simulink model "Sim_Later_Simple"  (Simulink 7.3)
settings: Solver=ode45  StartTime=0.0  StopTime=20  RelTol=1e-3
InitFcn:
  | init
StartFcn:
  | init
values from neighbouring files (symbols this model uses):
  d2r = pi/180    (= 0.0174532925199)    [init.m]    (also in robust.m)
  r2d = 180/pi    (= 57.2957795131)    [init.m]    (also in robust.m)
undefined symbols (not defined in the file or in its folder): Als, Bls, Cls, Dls, Kmix, Kpr

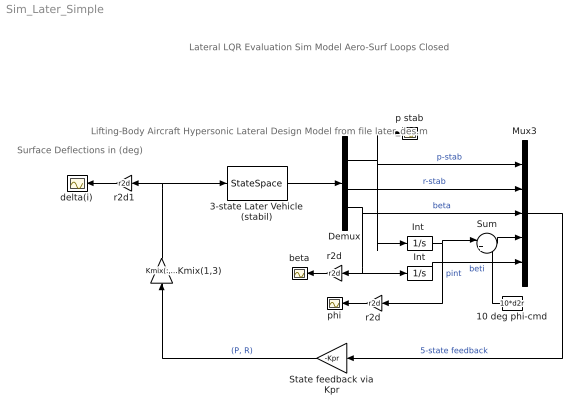
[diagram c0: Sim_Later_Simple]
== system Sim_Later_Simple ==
  note: Lateral LQR Evaluation Sim Model Aero-Surf Loops Closed
  note: Surface Deflections in (deg)
  note: Lifting-Body Aircraft Hypersonic Lateral Design Model from file later_des.m
  10 deg phi-cmd : Constant  Value=10*d2r  OutDataType=sfix(16)  OutScaling=2^0
  3-state Later Vehicle (stabil) : StateSpace  A=Als  B=Bls  C=Cls  D=Dls
  Demux : Demux  Outputs=3
  Int : Integrator
  "Int " : Integrator
  Kmix(1,3) : Gain  Gain=Kmix(:,[1,3])  Multiplication=Matrix(K*u)  ParameterDataType=sfix(16)  ParameterScaling=2^0  OutDataType=sfix(16)  OutScaling=2^0
  Mux3 : Mux  Inputs=5
  State feedback via Kpr : Gain  Gain=-Kpr  Multiplication=Matrix(K*u)  ParameterDataType=sfix(16)  ParameterScaling=2^0  OutDataType=sfix(16)  OutScaling=2^0
  Sum : Sum  Inputs=|+-  OutDataType=sfix(16)  OutScaling=2^0
  beta : Scope
  delta(i) : Scope
  p stab : Scope
  phi : Scope
  r2d : Gain  Gain=r2d  ParameterDataType=sfix(16)  ParameterScaling=2^0  OutDataType=sfix(16)  OutScaling=2^0
  "r2d " : Gain  Gain=r2d  ParameterDataType=sfix(16)  ParameterScaling=2^0  OutDataType=sfix(16)  OutScaling=2^0
  r2d1 : Gain  Gain=r2d  ParameterDataType=sfix(16)  ParameterScaling=2^0  OutDataType=sfix(16)  OutScaling=2^0
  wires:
  3-state Later Vehicle (stabil)/1 -> Demux/1
  Demux/1 -> Mux3/1, p stab/1, "Int "/1  "p-stab"
  Demux/2 -> Mux3/2  "r-stab"
  Demux/3 -> Mux3/3, r2d/1, Int/1  "beta"
  r2d/1 -> beta/1
  Mux3/1 -> State feedback via Kpr/1  "5-state feedback"
  "Int "/1 -> Sum/1, "r2d "/1  "pint"
  10 deg phi-cmd/1 -> Sum/2
  Sum/1 -> Mux3/4
  Int/1 -> Mux3/5  "beti"
  "r2d "/1 -> phi/1
  State feedback via Kpr/1 -> Kmix(1,3)/1  "(P, R)"
  Kmix(1,3)/1 -> 3-state Later Vehicle (stabil)/1, r2d1/1
  r2d1/1 -> delta(i)/1
